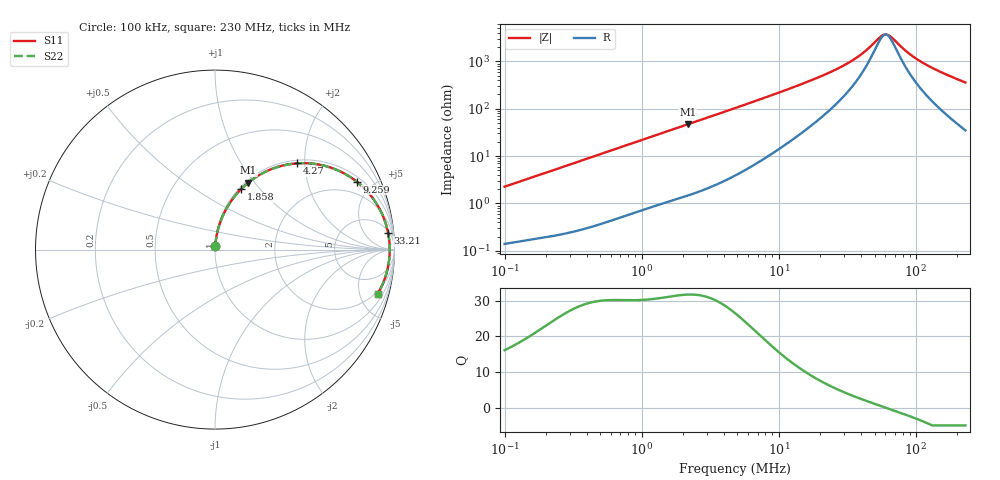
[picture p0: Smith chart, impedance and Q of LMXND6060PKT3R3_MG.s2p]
! LMXND6060PKT3R3_MG  S-PARAMETER MODEL  ( General Type )
! Model Generated by TAIYO YUDEN Corporation (https://www.yuden.co.jp/en/)
! Version 1.0
! TAIYO YUDEN Control No. 191025NI43SB-FBB
! Copyright(c) 2019 TAIYO YUDEN CO.,LTD. All Rights Reserved.
! Product Description (link to TY-COMPAS)
! https://ds.yuden.co.jp/TYCOMPAS/or/detail?pn=LMXND6060PKT3R3NMG&u=M
! Products Name : Inductors
! Characteristics :
!  Inductance : 3.3 uH , SRF(min) : 41 MHz , DC Resistance(max) : 0.09 Ohm
!  Rated Current : Saturation :2500 mA , Temp Rise : 2000 mA (40 degC)
!  Case Size : 6.0 x 6.0 / 0.236 x 0.236 [mm/inch] , Thickness : 1.4 / 0.055 [mm/inch]
!  (Conditions: Temperature = 25 degC , DC Bias Current/Voltage = 0A / 0V)
! External Node Assignments :
!  1  o---GGG---o  2
! GND o---------o GND
! Frequency Range : 0.1MHz  -  229.966873MHz  [ 402 STEP ]
# MHz S RI R 50
! Freq[MHz].  S11 Real  S11 Imag  S21 Real  S21 Imag  S12 Real  S12 Imag  S22 Real  S22 Imag
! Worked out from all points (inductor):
!   401 points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, 100 kHz to 230 MHz, reference 50 ohm
!   read as one part in series: L = 3.57 uH near 103.9 kHz
!   highest Q = 31.8 at 2.169 MHz (marker M1), where L = 3.41 uH
!   self-resonance near 60.25 MHz
!   S11 on the Smith chart (normalised r, x): 100 kHz: 1.00, +0.05; 1.858 MHz: 1.03, +0.80; 4.27 MHz: 1.07, +1.83; 9.259 MHz: 1.24, +4.02; 33.21 MHz: 6, +19; 230 MHz: 1.70, -7.15
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0.1  0.00191 0.0225  0.9981 -0.0225  0.9981 -0.0225  0.00191 0.0225
0.365661  0.00923 0.0798  0.9908 -0.0798  0.9908 -0.0798  0.00923 0.0798
0.719821  0.029 0.152  0.971 -0.152  0.971 -0.152  0.029 0.152
1.337081  0.0843 0.262  0.9157 -0.262  0.9157 -0.262  0.0843 0.262
1.857927  0.1454 0.337  0.8546 -0.337  0.8546 -0.337  0.1454 0.337
2.169012  0.1857 0.3735  0.8143 -0.3735  0.8143 -0.3735  0.1857 0.3735
2.956164  0.2923 0.439  0.7077 -0.439  0.7077 -0.439  0.2923 0.439
4.269801  0.4572 0.4807  0.5428 -0.4807  0.5428 -0.4807  0.4572 0.4807
4.889189  0.5229 0.4808  0.4771 -0.4808  0.4771 -0.4808  0.5229 0.4808
6.535807  0.6578 0.4522  0.3422 -0.4522  0.3422 -0.4522  0.6578 0.4522
9.259215  0.7888 0.3793  0.2112 -0.3793  0.2112 -0.3793  0.7888 0.3793
17.53523  0.9206 0.2196  0.0794 -0.2196  0.0794 -0.2196  0.9206 0.2196
24.842  0.9511 0.1453  0.0489 -0.1453  0.0489 -0.1453  0.9511 0.1453
33.20848  0.9646 0.0925  0.0354 -0.0925  0.0354 -0.0925  0.9646 0.0925
41.8889  0.9705 0.0547  0.0295 -0.0547  0.0295 -0.0547  0.9705 0.0547
55.99656  0.9735 0.0108  0.0265 -0.0108  0.0265 -0.0108  0.9735 0.0108
60.50315  0.9736 -0.000622  0.0264 0.000622  0.0264 0.000622  0.9736 -0.000622
64.11956  0.9735 -0.00921  0.0265 0.00921  0.0265 0.00921  0.9735 -0.00921
85.71424  0.9708 -0.053  0.0292 0.053  0.0292 0.053  0.9708 -0.053
108.1192  0.9651 -0.0907  0.0349 0.0907  0.0349 0.0907  0.9651 -0.0907
153.1715  0.9484 -0.1547  0.0516 0.1547  0.0516 0.1547  0.9484 -0.1547
229.9669  0.9075 -0.2449  0.0925 0.2449  0.0925 0.2449  0.9075 -0.2449
